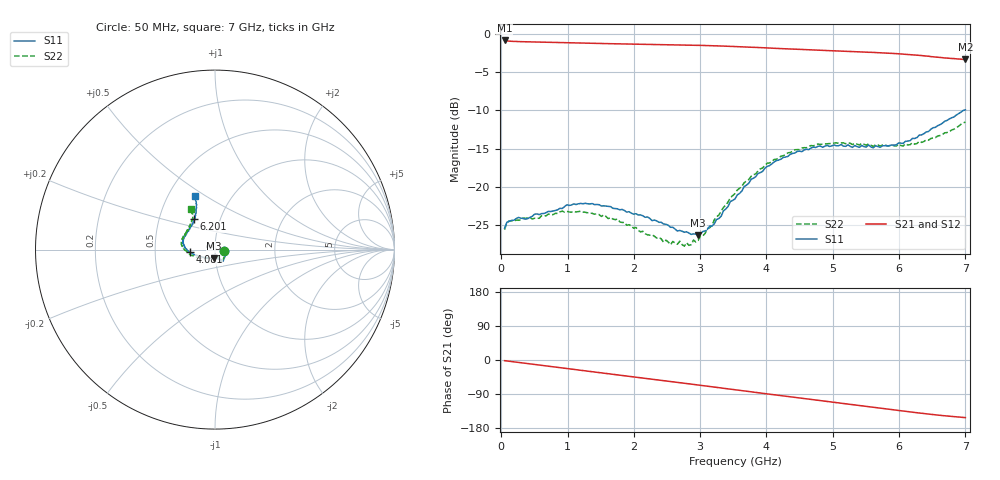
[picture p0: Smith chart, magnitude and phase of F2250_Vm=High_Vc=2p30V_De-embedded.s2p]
! Integrated Device Technology
! Corporate Headquarters
! 6024 Silver Creek Valley Road
! San Jose, CA 95138  USA
! Phone:  1-408-284-8200
! Toll Free:  1-800-223-1366
! Webpage:  http://www.idt.com/
! Timing and RF Division
! 515 Groton Road, Suite 102
! Westford, MA 01886-6024
! Device:  F2250
! Description: Voltage Variable RF Attenuator
! Frequency:  50.0 -  6000.00 MHz
! Package:  3x3 mm Thin QFN Plastic Package: 16 pin
! Ports:  2 RF, 3 DC
!  Pin  1  = GND
!  Pin  2  = NC
!  Pin  3  = RF1  = Port 1
!  Pin  4  = NC
!  Pin  5  = GND
!  Pin  6  = GND
!  Pin  7  = GND
!  Pin  8  = GND
!  Pin  9  = NC
!  Pin 10  = RF2  = Port 2
!  Pin 11  = NC
!  Pin 12  = GND
!  Pin 13  = GND
!  Pin 14  = VCNTRL
!  Pin 15  = VDD
!  Pin 16  = VMODE
! Vcntrl:  2.300 Volts
! Vmode:  +3.300 Volts
! Vdd:  +3.30  Volts
! Current:  1.316 mA
! Data:  The device was measured on a the F2250 evaluation board which has
!  individual transmission lines to the RF pins.  Data was collected
!  using a calibrated network analyzer.  The evaluation board was
!  de-embedded using a TRL calibration technique.
!  The reference plane is the edge of the package pin.
! Misc:  SN 10
!  Action Tracker AT0258
! Date Measured:  2014-11-26
! Date:  2015-10-15  MJV
! Note:
!  Integrated Device Technology supplies this data as a sample of measured
!  data at the package pin for this product.  Your particular data for this
!  product may vary.
!  Data was taken at 25 degrees C.
!  Integrated Device Technology reserves the right to change this data at anytime.
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# GHz S dB R 50
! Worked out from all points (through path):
!   201 points, 50 MHz to 7 GHz, reference 50 ohm
!   highest |S21| = -0.91 dB at 50 MHz (marker M1); lowest = -3.4 dB at 7 GHz (marker M2)
!   group delay of S21, straight-line fit = 61.2 ps
!   lowest |S11| = -26.3 dB at 2.969 GHz (marker M3), VSWR 1.10, Z = 49.3 - j4.76 ohm
!   |S11| at or under -10 dB: start of sweep to 6.981 GHz
!   |S22| runs from -27.7 to -11.5 dB; largest |S21 - S12| = 0.0019
!   S11 on the Smith chart (normalised r, x): 50 MHz: 1.11, -0.02; 4.081 GHz: 0.75, -0.02; 6.201 GHz: 0.75, +0.27; 7 GHz: 0.68, +0.45
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0.05  -25.39 -10.3  -0.91 -1.8  -0.91 -1.8  -25.56 -10.7
0.1195  -24.49 -10.0  -1.00 -3.2  -1.00 -3.2  -24.44 -8.7
0.91875  -22.82 -49.3  -1.19 -21.0  -1.19 -21.1  -23.15 -50.5
1.2315  -22.20 -57.0  -1.25 -27.9  -1.25 -27.9  -23.27 -61.0
1.75275  -22.85 -64.0  -1.35 -39.1  -1.35 -39.1  -24.19 -67.6
2.37825  -24.62 -63.8  -1.44 -52.8  -1.44 -52.8  -26.57 -67.2
2.552  -25.26 -68.6  -1.46 -56.7  -1.46 -56.7  -27.54 -73.7
2.691  -25.67 -76.4  -1.49 -59.8  -1.49 -59.8  -27.07 -81.3
2.7605  -25.91 -78.6  -1.50 -61.3  -1.50 -61.3  -27.72 -85.7
2.969  -26.29 -96.2  -1.54 -66.0  -1.54 -66.0  -26.99 -104.9
3.21225  -24.82 -126.3  -1.60 -71.5  -1.60 -71.5  -24.30 -129.9
3.4555  -21.90 -147.2  -1.67 -77.0  -1.67 -77.0  -21.39 -145.2
3.525  -21.56 -151.6  -1.70 -78.5  -1.70 -78.6  -20.86 -148.4
3.76825  -19.01 -163.9  -1.79 -84.0  -1.79 -84.0  -18.62 -159.4
4.081  -17.00 -175.1  -1.92 -91.0  -1.91 -91.0  -16.67 -171.2
4.4285  -15.58 176.5  -2.05 -98.6  -2.05 -98.6  -15.15 178.8
4.7065  -14.81 169.5  -2.14 -104.8  -2.15 -104.8  -14.65 173.1
5.054  -14.65 161.4  -2.28 -112.5  -2.27 -112.5  -14.25 166.0
5.85325  -14.62 135.5  -2.57 -130.0  -2.57 -130.1  -14.65 147.3
6.20075  -13.67 123.9  -2.78 -137.7  -2.78 -137.8  -14.24 138.3
6.54825  -12.23 115.9  -3.05 -144.7  -3.06 -144.9  -13.57 126.9
7  -9.95 111.0  -3.38 -152.1  -3.39 -152.2  -11.54 120.7
